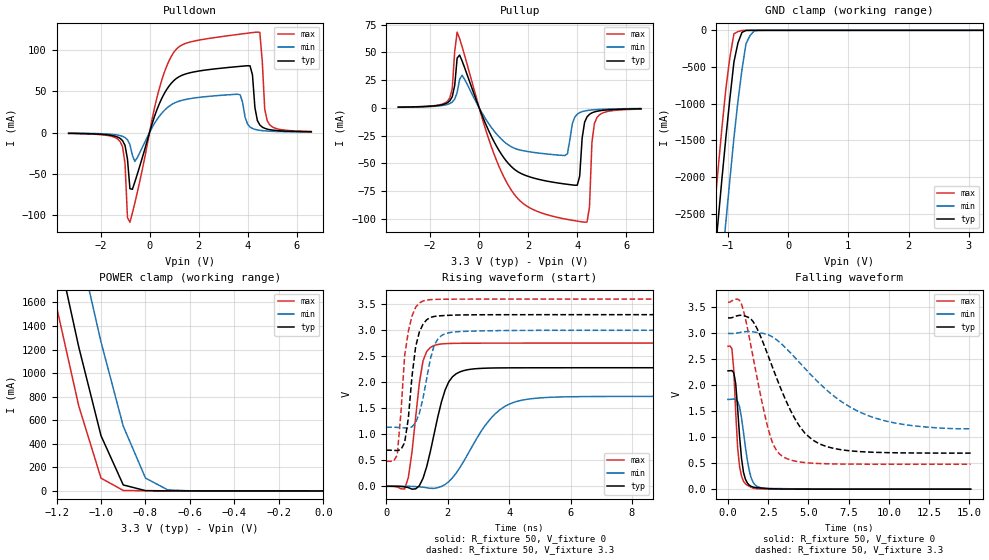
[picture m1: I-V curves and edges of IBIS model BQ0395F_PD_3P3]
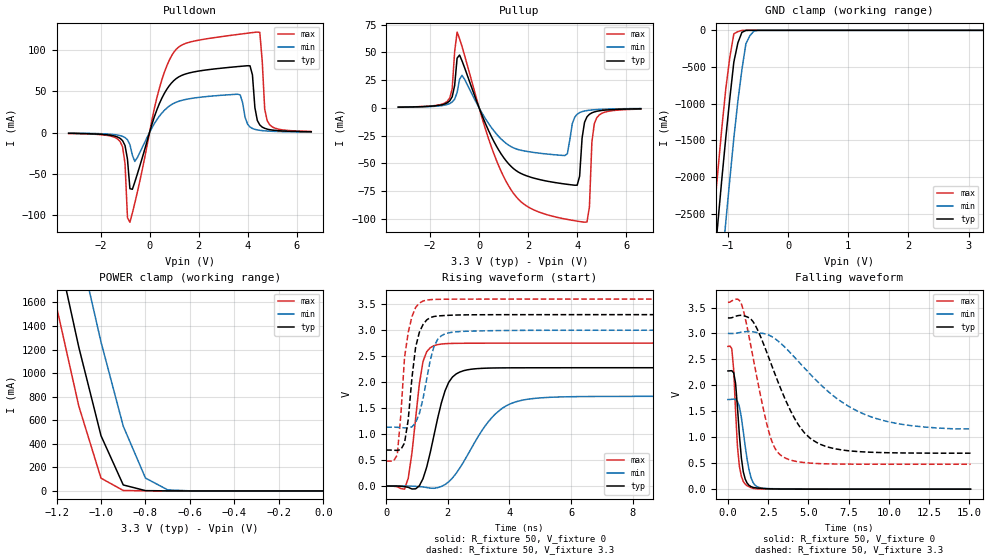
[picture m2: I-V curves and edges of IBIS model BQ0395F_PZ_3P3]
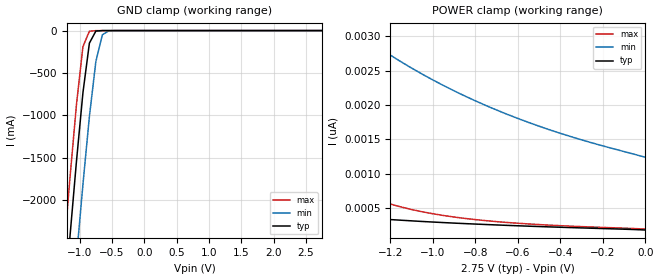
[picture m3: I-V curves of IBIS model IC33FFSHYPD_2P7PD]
[IBIS Ver]   3.2
[File Name]   sprm738.ibs
[File Rev]   1.0
[Date]   February 11, 2008
[Source]   File originated at Texas Instruments
[Copyright]   (c) 2008, Texas Instruments Inc.
[Component]   f741804rsh
[Manufacturer] Texas Instruments
[Package]
| Variable   Typ   Min   Max
R_pkg   0.286   0.114   0.385
L_pkg   1.59e-09   1.25e-09   1.98e-09
C_pkg   2.6e-12   0.146e-12   0.556e-12
[Pin] signal_name   model_name   R_pin   L_pin   C_pin
1	GP_IO[22]	BQ0393F   0.31	1.60E-09	5.34E-13
2	GP_IO[23]	BQ0393F   0.28	1.54E-09	1.93E-13
3	VDD   NC   0.28	1.52E-09	1.91E-13
4	VSS   NC   0.29	1.49E-09	1.93E-13
5	XRSn   BC3350BFODHYPU 	0.27	1.42E-09	1.92E-13
6	TRSTn   IC33FFSHYPD   0.27	1.41E-09	1.89E-13
7	ADCINA7   NC   0.26	1.37E-09	1.92E-13
8	ADCINA6   NC   0.26	1.41E-09	5.38E-13
9	ADCINA4   NC   0.28	1.48E-09	5.41E-13
10	ADCINA3   NC   0.31	1.60E-09	5.43E-13
11	ADCINA2   NC   0.33	1.70E-09	4.88E-13
12	ADCINA1   NC   0.36	1.87E-09	5.56E-13
13	ADCINA0   NC   0.31	1.61E-09	4.69E-13
14	VDDAFL   NC   0.32	1.62E-09	3.45E-13
15	VSSA   NC   0.32	1.64E-09	5.02E-13
16	ADCINB1   NC   0.37	1.92E-09	2.26E-13
17	ADCINB2   NC   0.21	1.74E-09	2.70E-13
18	ADCINB3   NC   0.19	1.62E-09	2.80E-13
19	ADCINB4   NC   0.18	1.49E-09	2.70E-13
20	ADCINB6   NC   0.39	1.98E-09	2.45E-13
21	ADCINB7   NC   0.35	1.78E-09	3.53E-13
22	GP_IO[31]	BQ0393F   0.33	1.75E-09	2.33E-13
23	GP_IO[30]	BQ0393F   0.17	1.38E-09	2.50E-13
24	GP_IO[29]	BQ0395F   0.31	1.59E-09	2.25E-13
25	VSS   NC   0.31	1.61E-09	2.23E-13
26	VDDSFL   NC   0.32	1.63E-09	2.24E-13
27	TEST2   NC   0.17	1.39E-09	2.50E-13
28	GP_IO[28]	BQ0395F   0.34	1.81E-09	2.83E-13
29	GP_IO[18]	BQ0395F   0.17	1.40E-09	2.49E-13
30	GP_IO[17]	BQ0395F   0.34	1.76E-09	1.53E-13
31	GP_IO[16]	BQ0395F   0.31	1.67E-09	1.62E-13
32	GP_IO[12]	BQ0393F   0.29	1.56E-09	1.49E-13
33	GP_IO[7]	BQ0393F   0.27	1.49E-09	1.46E-13
34	GP_IO[6]	BQ0393F   0.27	1.47E-09	1.46E-13
35	X2   NC   0.27	1.47E-09	1.46E-13
36	X1   NC   0.27	1.41E-09	1.70E-13
37	VSS   NC   0.28	1.46E-09	1.72E-13
38	VDD   NC   0.30	1.59E-09	1.73E-13
39	GP_IO[19]	BC3325CFHYPU 	0.31	1.67E-09	1.77E-13
40	GP_IO[38]	BC3350AFHYPU 	0.12	1.35E-09	2.25E-13
41	GP_IO[37]	BC3325CFHYPU 	0.32	1.67E-09	1.73E-13
42	GP_IO[35]	BC3350AFHYPU 	0.32	1.66E-09	1.69E-13
43	GP_IO[36]	BC3325CFHYPU 	0.32	1.69E-09	2.20E-13
44	GP_IO[5]	BQ0393F   0.32	1.70E-09	1.76E-13
45	GP_IO[4]	BQ0393F   0.33	1.74E-09	1.78E-13
46	GP_IO[3]	BQ0393F   0.32	1.71E-09	1.77E-13
47	GP_IO[2]	BQ0483F   0.33	1.73E-09	1.70E-13
48	GP_IO[1]	BQ0483F   0.32	1.72E-09	1.73E-13
49	GP_IO[0]	BQ0393F   0.32	1.70E-09	1.79E-13
50	VDDSFL   NC   0.31	1.60E-09	1.79E-13
51	VSS   NC   0.11	1.25E-09	3.30E-13
52	VDD   NC   0.12	1.28E-09	3.35E-13
53	VREGENZ   NC   0.33	1.69E-09	2.83E-13
54	GP_IO[34]	BC3350AFHYPU 	0.32	1.63E-09	2.77E-13
55	GP_IO[20]	BQ0393F   0.32	1.63E-09	2.77E-13
56	GP_IO[21]	BQ0393F   0.33	1.66E-09	2.17E-13
| End of package information
[Component]   BQ0395F
[Manufacturer]   Texas Instruments
[Package]
|  variable   typ   min   max
R_pkg   0   0   0
L_pkg   0   0   0
C_pkg   0   0   0
[Pin]   signal_name   model_name   R_pin   L_pin   C_pin
VSS   VSS   GND
VDDS   VDDS   POWER
PAD   PAD   BQ0395F
[Model Selector] BQ0395F
BQ0395F_PD_3P3  Cell operated at 3.3(nom)
|BQ0395F_PD_3P3; PULLDOWN_ON
BQ0395F_PZ_3P3  Cell operated at 3.3(nom)
[Component]   IC33FFSHYPD
[Manufacturer]   Texas Instruments.
[Package]
| variable   typ   min   max
R_pkg   0.000   0.000   0.000
L_pkg   0.000H   0.000H   0.000H
C_pkg   0.000F   0.000F   0.000F
[Pin]  signal_name   model_name   R_pin   L_pin   C_pin
PAD   PAD   IC33FFSHYPD_3P3PD
| Y   Y   dummy
VSS   VSS   GND
VDDS   VDDS   POWER
[Model Selector]  IC33FFSHYPD
IC33FFSHYPD_2P7PD   cell with PI=0 and VDDS as 2.75(typ)
IC33FFSHYPD_2P7PDZ   cell with PI=1 and VDDS as 2.75(typ)
IC33FFSHYPD_3P3PD   cell with PI=0 and VDDS as 3.3(typ)
IC33FFSHYPD_3P3PDZ   cell with PI=1 and VDDS as 3.3(typ)
|   Component IC33FFSHYPU
[Component]   BC3350BFODHYPU
[Manufacturer]   Texas Instruments.
[Package]
| variable   typ   min   max
R_pkg   0.000   0.000   0.000
L_pkg   0.000H   0.000H   0.000H
C_pkg   0.000F   0.000F   0.000F
[Pin]  signal_name   model_name   R_pin   L_pin   C_pin
PAD   PAD   BC3350BFODHYPU_3P3PU
| A   A   dummy
| GZ   GZ   dummy
| Y   Y   dummy
VSSS   VSSS   GND
VDDS   VDDS   POWER
[Model Selector]   BC3350BFODHYPU
BC3350BFODHYPU_2P5PU   cell   VDDS=2.75(TYP)
BC3350BFODHYPU_2P5PZ   cell   VDDS=2.75(TYP)
BC3350BFODHYPU_3P3PU   cell   VDDS=3.3(TYP)
BC3350BFODHYPU_3P3PZ   cell   VDDS=3.3(TYP)
|   Component IC33FFSHY
[Component]   BC3350AFHYPU
[Manufacturer]   Texas Instruments.
[Package]
| variable   typ   min   max
R_pkg   0.000   0.000   0.000
L_pkg   0.000H   0.000H   0.000H
C_pkg   0.000F   0.000F   0.000F
[Pin]  signal_name   model_name   R_pin   L_pin   C_pin
PAD   PAD   BC3350AFHYPU_3P3PU
| A   A   dummy
| GZ   GZ   dummy
| Y   Y   dummy
VSSS   VSSS   GND
VDDS   VDDS   POWER
[Model Selector]  BC3350AFHYPU
BC3350AFHYPU_2P5PU   cell   VDDS=2.5V(typ)  PI=0
BC3350AFHYPU_2P5PUZ  cell   VDDS=2.5V(typ)  PI=1
BC3350AFHYPU_3P3PU   cell   VDDS=3.3V(typ)  PI=0
BC3350AFHYPU_3P3PUZ  cell   VDDS=3.3V(typ)  PI=1
|   Component OC3325CF
[Component]   BC3325CFHYPU
[Manufacturer]   Texas Instruments.
[Package]
| variable   typ   min   max
R_pkg   0.000   0.000   0.000
L_pkg   0.000H   0.000H   0.000H
C_pkg   0.000F   0.000F   0.000F
[Pin]  signal_name   model_name   R_pin   L_pin   C_pin
PAD   PAD   BC3325CFHYPU_3P3PU
| A   A   dummy
| GZ   GZ   dummy
| Y   Y   dummy
VSSS   VSSS   GND
VDDS   VDDS   POWER
[Model Selector]   BC3325CFHYPU
BC3325CFHYPU_2P5PU   cell  VDDS=2.75(TYP)  PI=0
BC3325CFHYPU_2P5PUZ   cell  VDDS=2.75(TYP)  PI=1
BC3325CFHYPU_3P3PU   cell  VDDS=3.3(TYP)  PI=0
BC3325CFHYPU_3P3PUZ   cell  VDDS=3.3(TYP)  PI=1
|   Component BC3350AFHYPU
[Component]   BQ0483F
[Manufacturer]   Texas Instruments
[Package]
|  variable   typ   min   max
R_pkg   0   0   0
L_pkg   0   0   0
C_pkg   0   0   0
[Pin]   signal_name   model_name   R_pin   L_pin   C_pin
VSS   VSS   GND
VDDS   VDDS   POWER
PAD   PAD   BQ0483F
[Model Selector] BQ0483F
BQ0483F_PD_3P3  Cell operated at 3.3(nom)
|BQ0483F_PD_3P3; PULLDOWN_ON
BQ0483F_PZ_3P3  Cell operated at 3.3(nom)
[Component]   BQ0393F
[Manufacturer]   Texas Instruments
[Package]
|  variable   typ   min   max
R_pkg   0   0   0
L_pkg   0   0   0
C_pkg   0   0   0
[Pin]   signal_name   model_name   R_pin   L_pin   C_pin
VSS   VSS   GND
VDDS   VDDS   POWER
PAD   PAD   BQ0393F
[Model Selector] BQ0393F
BQ0393F_PD_3P3  Cell operated at 3.3(nom)
|BQ0393F_PD_3P3; PULLDOWN_ON
BQ0393F_PZ_3P3  Cell operated at 3.3(nom)
| Models and submodels in the file (22): BQ0395F_PD_3P3 (I/O), BQ0395F_PZ_3P3 (I/O), IC33FFSHYPD_2P7PD (Input), IC33FFSHYPD_2P7PDZ (Input), IC33FFSHYPD_3P3PD (Input), IC33FFSHYPD_3P3PDZ (Input), BC3350BFODHYPU_2P5PU (I/O_open_drain), BC3350BFODHYPU_2P5PZ (I/O_open_drain), BC3350BFODHYPU_3P3PU (I/O_open_drain), BC3350BFODHYPU_3P3PZ (I/O_open_drain), BC3350AFHYPU_2P5PU (I/O), BC3350AFHYPU_2P5PUZ (I/O), BC3350AFHYPU_3P3PU (I/O), BC3350AFHYPU_3P3PUZ (I/O), BC3325CFHYPU_2P5PU (I/O), BC3325CFHYPU_2P5PUZ (I/O), BC3325CFHYPU_3P3PU (I/O), BC3325CFHYPU_3P3PUZ (I/O), BQ0483F_PD_3P3 (I/O), BQ0483F_PZ_3P3 (I/O), BQ0393F_PD_3P3 (I/O), BQ0393F_PZ_3P3 (I/O)
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|BQ0395F_PZ_3P3; PULLDOWN_OFF
|   Model Cell BQ0395F_PD_3P3
|BQ0395F_PD_3P3
[Model]   BQ0395F_PD_3P3
Model_type   I/O
Polarity   Non-Inverting
Enable   Active-Low
Vinl =  1.15
Vinh =  1.65
Cref =  15.0001pF
Rref =  101.0000M
Vref =  0V
Vmeas =  1.65
C_comp   1.2p   1.2p   1.2p
[Model Spec]
Vinl   1.15   1.05   1.15
Vinh   1.65   1.65   1.65
[Temperature Range]   25   125   -40
[Voltage Range]   3.3   3   3.6
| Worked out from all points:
|   slope of the pulldown table from 0 to 0.495 V, typ, clamps not added: 12 ohm
|   slope of the pullup table from 0 to 0.495 V, typ, clamps not added: 19.4 ohm
|   GND clamp passes 1 mA (typ) near -0.66 V on its own axis
|   POWER clamp passes 1 mA (typ) near -0.72 V on its own axis
|   rising waveform, R_fixture 50, V_fixture 0: 20-80 % time 553ps typ, 1.15ns min, 327ps max; typ from 0.001 V to 2.28 V
|   rising waveform, R_fixture 50, V_fixture 3.3: 20-80 % time 302ps typ, 400ps min, 286ps max; typ from 0.695 V to 3.3 V
|   falling waveform, R_fixture 50, V_fixture 0: 20-80 % time 372ps typ, 499ps min, 308ps max; typ from 2.28 V to 0.001 V
|   falling waveform, R_fixture 50, V_fixture 3.3: 20-80 % time 2.21ns typ, 4.03ns min, 1.26ns max; typ from 3.3 V to 0.695 V
[POWER_clamp]
|   voltage   I(typ)   I(min)   I(max)
-3.3V     22.47A     23.26A     22.03A
-1.233V   2.386A     3.273A     1.866A
-1.2V     2.084A     2.97A      1.564A
-1.167V   1.796A     2.677A     1.283A
-1.133V   1.509A     2.384A     1.002A
-1.067V   970.3mA    1.815A     516.3mA
-1.033V   719.4mA    1.539A     312.3mA
-1V       468.5mA    1.264A     108.3mA
-900mV    50.9mA     550mA      3.945mA
-800mV    2.599mA    109.2mA    1.152mA
-700mV    531.1uA    8.818mA    336.1uA
0V        279.6pA    1.919nA    325pA
[Pulldown]
|   voltage   I(typ)   I(min)   I(max)
-3.3V     -988.5uA   -708.3uA   -1.157mA
-1.2V     -7.098mA   -3.712mA   -10.91mA
-800mV    -68.22mA   -14.66mA   -108.9mA
-600mV    -60.07mA   -35.15mA   -85.64mA
300mV     27.57mA    15.61mA    42.26mA
1V        63.3mA     35.61mA    97.86mA
3.7V      80.34mA    45.74mA    119.5mA
4.1V      80.98mA    6.702mA    121mA
4.4V      14.6mA     3.158mA    122mA
4.5V      9.15mA     2.669mA    121.7mA
4.8V      4.146mA    1.814mA    14.51mA
6.6V      929.5uA    610.9uA    1.29mA
[Pullup]
|   voltage   I(typ)   I(min)   I(max)
-3.3V     680.2uA    582.8uA    724.9uA
-1.3V     4.616mA    3.102mA    5.939mA
-900mV    44.89mA    13.88mA    68.33mA
600mV     -30.17mA   -20.61mA   -41.26mA
1.7V      -59mA      -38.13mA   -84.39mA
3.5V      -68.55mA   -42.86mA   -100.1mA
4V        -69.63mA   -5.654mA   -102mA
4.3V      -12.95mA   -2.78mA    -103mA
4.5V      -5.735mA   -2.056mA   -89.2mA
4.6V      -4.432mA   -1.817mA   -30.89mA
4.8V      -3.028mA   -1.473mA   -8.825mA
6.6V      -767.6uA   -538uA     -1.05mA
[GND_clamp]
|   voltage   I(typ)   I(min)   I(max)
-3.3V     -23.4A     -24.5A     -22.76A
-1.3V     -3.866A    -5.045A    -3.159A
-1.233V   -3.247A    -4.425A    -2.54A
-1.167V   -2.635A    -3.811A    -1.931A
-1.033V   -1.46A     -2.609A    -794.5mA
-966.7mV  -926.2mA   -2.032A    -365.7mA
-900mV    -431.8mA   -1.469A    -47.48mA
-833.3mV  -172mA     -967.1mA   -17.77mA
-766.7mV  -28.5mA    -538.6mA   -2.104mA
-700mV    -1.454mA   -183.8mA   -472.2uA
-566.7mV  -175.9uA   -11.4mA    -230.7uA
3.233V    -8.123uA   19.88uA    -59.92uA
[Ramp]
| variable   typ   min   max
dV/dt_f   2.125235/3.393203n   1.522792/6.529444n   2.546199/1.871013n
dV/dt_r   1.870375/0.8633114n   1.417739/1.795571n   2.257927/0.4923715n
R_load = 50
[Rising Waveform]
R_fixture = 50
V_fixture = 0
V_fixture_min = 0
V_fixture_max = 0
|   time   V(typ)   V(min)   V(max)
0s        1.011mV    996.9uV    1.133mV
600ps     -10.22mV   1.405mV    -51.04mV
720ps     -23.4mV    678.7uV    169.5mV
1.2ns     155.9mV    -16.37mV   2.416V
1.556ns   996.6mV    -39.43mV   2.707V
1.916ns   1.849V     34.62mV    2.743V
2.276ns   2.164V     253.6mV    2.749V
3.44ns    2.275V     1.329V     2.753V
4.344ns   2.279V     1.646V     2.753V
15.09ns   2.28V      1.73V      2.754V
[Rising Waveform]
R_fixture = 50
V_fixture = 3.3
V_fixture_min = 3
V_fixture_max = 3.6
|   time   V(typ)   V(min)   V(max)
0s        694.6mV    1.135V     482.1mV
360ps     687.7mV    1.134V     601.7mV
480ps     707.3mV    1.129V     1.417V
600ps     840mV      1.123V     2.509V
720ps     1.306V     1.122V     2.977V
960ps     2.69V      1.227V     3.444V
1.2ns     3.117V     1.697V     3.564V
1.556ns   3.265V     2.698V     3.593V
2.036ns   3.288V     2.952V     3.598V
15.09ns   3.3V       3V         3.6V
[Falling Waveform]
R_fixture = 50
V_fixture = 0
V_fixture_min = 0
V_fixture_max = 0
|   time   V(typ)   V(min)   V(max)
0s        2.28V      1.73V      2.753V
240ps     2.285V     1.734V     2.71V
360ps     2.243V     1.738V     2.295V
480ps     2.031V     1.73V      1.476V
720ps     1.017V     1.582V     435.1mV
960ps     332.5mV    1.104V     155.7mV
1.2ns     120.6mV    564.9mV    75.69mV
1.556ns   42.01mV    135.6mV    22.21mV
2.156ns   20.25mV    22.83mV    5.408mV
15.09ns   1.097mV    1.119mV    1.182mV
[Falling Waveform]
R_fixture = 50
V_fixture = 3.3
V_fixture_min = 3
V_fixture_max = 3.6
|   time   V(typ)   V(min)   V(max)
0s        3.3V       3V         3.599V
840ps     3.35V      3.025V     3.566V
1.556ns   3.23V      3.032V     2.552V
2.516ns   2.556V     2.972V     1.143V
2.876ns   2.261V     2.911V     824.8mV
3.328ns   1.906V     2.798V     645.9mV
4.792ns   1.077V     2.324V     512.9mV
6.208ns   814.6mV    1.891V     489.5mV
9.672ns   706.3mV    1.325V     482.1mV
15.09ns   695.1mV    1.165V     482mV
|   Model Cell BQ0395F_PZ_3P3
|BQ0395F_PZ_3P3
[Model]   BQ0395F_PZ_3P3
Model_type   I/O
Polarity   Non-Inverting
Enable   Active-Low
Vinl =  1.15
Vinh =  1.65
Cref =  15.0001pF
Rref =  101.0000M
Vref =  0V
Vmeas =  1.65
C_comp   1.2p   1.2p   1.2p
[Model Spec]
Vinl   1.15   1.05   1.15
Vinh   1.65   1.65   1.65
[Temperature Range]   25   125   -40
[Voltage Range]   3.3   3   3.6
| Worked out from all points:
|   slope of the pulldown table from 0 to 0.495 V, typ, clamps not added: 12 ohm
|   slope of the pullup table from 0 to 0.495 V, typ, clamps not added: 19.3 ohm
|   GND clamp passes 1 mA (typ) near -0.68 V on its own axis
|   POWER clamp passes 1 mA (typ) near -0.73 V on its own axis
|   rising waveform, R_fixture 50, V_fixture 0: 20-80 % time 552ps typ, 1.15ns min, 326ps max; typ from 0 V to 2.28 V
|   rising waveform, R_fixture 50, V_fixture 3.3: 20-80 % time 301ps typ, 401ps min, 286ps max; typ from 0.693 V to 3.3 V
|   falling waveform, R_fixture 50, V_fixture 0: 20-80 % time 370ps typ, 499ps min, 306ps max; typ from 2.28 V to 0 V
|   falling waveform, R_fixture 50, V_fixture 3.3: 20-80 % time 2.2ns typ, 4.03ns min, 1.26ns max; typ from 3.3 V to 0.693 V
[POWER_clamp]
|   voltage   I(typ)   I(min)   I(max)
-3.3V     22.47A     23.26A     22.03A
-1.233V   2.386A     3.273A     1.866A
-1.2V     2.084A     2.97A      1.564A
-1.167V   1.796A     2.677A     1.283A
-1.133V   1.509A     2.384A     1.001A
-1.067V   970.3mA    1.815A     516.3mA
-1.033V   719.4mA    1.539A     312.3mA
-1V       468.5mA    1.264A     108.3mA
-900mV    50.85mA    550mA      3.793mA
-800mV    2.505mA    109.2mA    1.004mA
-700mV    437.8uA    8.783mA    205.6uA
0V        281.4pA    1.921nA    326.9pA
[Pulldown]
|   voltage   I(typ)   I(min)   I(max)
-3.3V     -988.5uA   -708.3uA   -1.157mA
-1.2V     -7.098mA   -3.712mA   -10.91mA
-800mV    -68.21mA   -14.66mA   -108.9mA
-600mV    -60.07mA   -35.15mA   -85.65mA
300mV     27.57mA    15.61mA    42.26mA
1V        63.3mA     35.61mA    97.86mA
3.7V      80.34mA    45.73mA    119.5mA
4.1V      80.98mA    6.702mA    121mA
4.4V      14.6mA     3.158mA    122mA
4.5V      9.15mA     2.669mA    121.7mA
4.8V      4.146mA    1.814mA    14.51mA
6.6V      929.5uA    610.9uA    1.29mA
[Pullup]
|   voltage   I(typ)   I(min)   I(max)
-3.3V     680.2uA    582.8uA    724.9uA
-1.3V     4.616mA    3.102mA    5.939mA
-900mV    44.88mA    13.88mA    68.33mA
600mV     -30.17mA   -20.61mA   -41.26mA
1.7V      -59mA      -38.13mA   -84.39mA
3.5V      -68.55mA   -42.86mA   -100.1mA
4V        -69.63mA   -5.654mA   -102mA
4.3V      -12.95mA   -2.78mA    -103mA
4.5V      -5.735mA   -2.056mA   -89.18mA
4.6V      -4.432mA   -1.817mA   -30.89mA
4.8V      -3.028mA   -1.473mA   -8.824mA
6.6V      -767.6uA   -538uA     -1.05mA
[GND_clamp]
|   voltage   I(typ)   I(min)   I(max)
-3.3V     -23.4A     -24.5A     -22.76A
-1.3V     -3.866A    -5.045A    -3.159A
-1.233V   -3.247A    -4.425A    -2.54A
-1.167V   -2.635A    -3.811A    -1.931A
-1.033V   -1.46A     -2.609A    -794.5mA
-966.7mV  -926.2mA   -2.032A    -365.6mA
-900mV    -431.8mA   -1.469A    -47.3mA
-833.3mV  -171.9mA   -967mA     -17.57mA
-766.7mV  -28.37mA   -538.6mA   -1.884mA
-700mV    -1.315mA   -183.8mA   -250.9uA
-566.7mV  -34.93uA   -11.32mA   -9.563uA
3.233V    268.2pA    281.8nA    247.8pA
[Ramp]
| variable   typ   min   max
dV/dt_f   2.127044/3.389099n   1.52501/6.522896n   2.547898/1.869267n
dV/dt_r   1.87233/0.8643675n   1.418387/1.796408n   2.260849/0.4926587n
R_load = 50
[Rising Waveform]
R_fixture = 50
V_fixture = 0
V_fixture_min = 0
V_fixture_max = 0
|   time   V(typ)   V(min)   V(max)
0s        -85.83uV   -72.94uV   -48.69uV
596ps     -11.15mV   351.6uV    -60.03mV
836ps     -56.28mV   -2.353mV   634.8mV
1.196ns   143.6mV    -17.49mV   2.401V
1.552ns   979.8mV    -43.14mV   2.703V
1.912ns   1.837V     29.22mV    2.741V
2.272ns   2.159V     246.3mV    2.747V
3.428ns   2.272V     1.317V     2.751V
4.328ns   2.277V     1.641V     2.752V
15.08ns   2.278V     1.727V     2.752V
[Rising Waveform]
R_fixture = 50
V_fixture = 3.3
V_fixture_min = 3
V_fixture_max = 3.6
|   time   V(typ)   V(min)   V(max)
0s        692.6mV    1.132V     480.3mV
360ps     685.7mV    1.131V     599.1mV
476ps     702.9mV    1.126V     1.367V
596ps     828.8mV    1.12V      2.476V
716ps     1.28V      1.119V     2.961V
956ps     2.675V     1.22V      3.439V
1.196ns   3.11V      1.681V     3.563V
1.552ns   3.265V     2.687V     3.592V
2.152ns   3.29V      2.962V     3.598V
15.08ns   3.3V       3V         3.6V
[Falling Waveform]
R_fixture = 50
V_fixture = 0
V_fixture_min = 0
V_fixture_max = 0
|   time   V(typ)   V(min)   V(max)
0s        2.278V     1.727V     2.751V
240ps     2.283V     1.732V     2.708V
360ps     2.241V     1.736V     2.291V
476ps     2.039V     1.728V     1.496V
716ps     1.028V     1.585V     434mV
956ps     333.3mV    1.11V      148.2mV
1.196ns   115.7mV    569.8mV    65.9mV
1.552ns   35.55mV    133.4mV    16.89mV
2.152ns   14.57mV    18.82mV    3.451mV
15.08ns   1.284uV    41.76uV    650.7nV
[Falling Waveform]
R_fixture = 50
V_fixture = 3.3
V_fixture_min = 3
V_fixture_max = 3.6
|   time   V(typ)   V(min)   V(max)
0s        3.3V       3V         3.599V
836ps     3.35V      3.024V     3.569V
1.552ns   3.232V     3.032V     2.555V
2.508ns   2.56V      2.973V     1.146V
2.98ns    2.174V     2.888V     758.9mV
3.428ns   1.828V     2.769V     622.7mV
4.776ns   1.079V     2.328V     511.4mV
6.192ns   813.2mV    1.893V     487.6mV
9.664ns   704.1mV    1.323V     480.2mV
15.08ns   693mV      1.162V     480.1mV
|   Model IC33FFSHYPD_2P7PD
[Model]   IC33FFSHYPD_2P7PD
Model_type   Input
Polarity   Non-Inverting
Vinl =   0.8250V
Vinh =   1.9250V
C_comp   2.1397pF   2.1767pF   2.7158pF
[Temperature Range]   25.0000   0.1250k   -40.0000
[Voltage Range]   2.7500V   2.5000V   3.0000V
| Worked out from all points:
|   GND clamp passes 1 mA (typ) near -0.66 V on its own axis
[GND_clamp]
| voltage   I(typ)   I(min)   I(max)
-2.75V    -17.91A    -19.01A    -17.27A
-1.25V    -3.342A    -4.502A    -2.646A
-1.15V    -2.424A    -3.58A     -1.732A
-1.05V    -1.541A    -2.68A     -871.7mA
-950mV    -732.7mA   -1.814A    -188.7mA
-850mV    -147.9mA   -1.014A    -7.752mA
-750mV    -6.009mA   -364.9mA   -798.7uA
-650mV    -206.4uA   -49.97mA   -59.18uA
-550mV    -9.486uA   -3.233mA   -2.615uA
2.75V     181.8pA    1.449nA    170.8pA
[POWER_clamp]
| voltage   I(typ)   I(min)   I(max)
-2.75V    1.398nA    9.161nA    24.63nA
-2.4V     922.6pA    6.884nA    9.415nA
-2V       612.2pA    5.001nA    3.237nA
-1.95V    584.8pA    4.808nA    2.846nA
-1.8V     512.9pA    4.278nA    1.955nA
-1.7V     472.6pA    3.961nA    1.538nA
-1.55V    421.6pA    3.534nA    1.095nA
-1.35V    367.1pA    3.045nA    729.7pA
-1.1V     315.3pA    2.541nA    480.7pA
-750mV    261.9pA    1.994nA    318pA
-400mV    222pA      1.589nA    244.9pA
0V        181.8pA    1.241nA    195.1pA
